ORGANIZATION_BLOCK "Power Supply Fault"
TITLE =
VERSION : 0.1


VAR_TEMP
  OB81_EV_CLASS : BYTE ;	//16#39, Event class 3, Entering event state, Internal fault event
  OB81_FLT_ID : BYTE ;	//16#XX, Fault identifcation code
  OB81_PRIORITY : BYTE ;	//26/28 (Priority of 1 is lowest)
  OB81_OB_NUMBR : BYTE ;	//81 (Organization block 81, OB81)
  OB81_RESERVED_1 : BYTE ;	//Reserved for system
  OB81_RESERVED_2 : BYTE ;	//Reserved for system
  OB81_MDL_ADDR : INT ;	//Reserved for system
  OB81_RESERVED_3 : BYTE ;	//Reserved for system
  OB81_RESERVED_4 : BYTE ;	//Reserved for system
  OB81_RESERVED_5 : BYTE ;	//Reserved for system
  OB81_RESERVED_6 : BYTE ;	//Reserved for system
  OB81_DATE_TIME : DATE_AND_TIME ;	//Date and time OB81 started
END_VAR
BEGIN
END_ORGANIZATION_BLOCK

